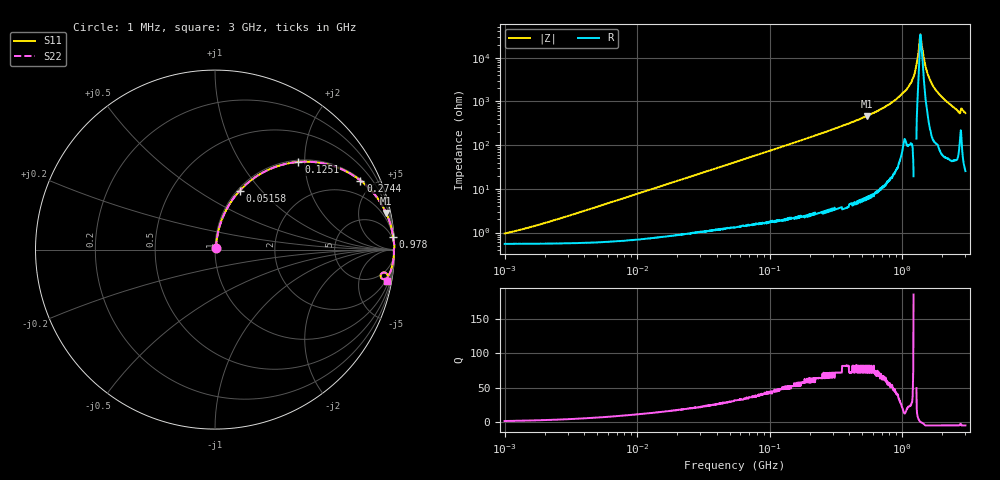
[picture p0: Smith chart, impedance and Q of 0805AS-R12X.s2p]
!s-Parameter Generated by FASTRON Sdn. Bhd.
!FASTRON P/N : 0805AS-R12X
!Keysight Technologies: E4991B_MY54100416_A.01.15
!Date: Mon Jun 15 12:52:09 2026
!Version  :Rev01  Mon Jun 15 12:52:09 2026
!Data & Calibration Information:
!Freq  S11  S21  S12  S22
!PortZ  Port1:50+j0  Port2:50+j0
!When reading reference impedance value at option line is always used.
! Remarks : This data is being provided solely for informational purposes.
# Hz S dB R 50
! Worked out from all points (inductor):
!   1601 points, 1 MHz to 3 GHz, reference 50 ohm
!   read as one part in series: L = 123 nH near 2.172 MHz
!   highest Q = 81.6 at 541.9 MHz (marker M1), where L = 137 nH
!   self-resonance near 1.374 GHz
!   S11 on the Smith chart (normalised r, x): 1 MHz: 1.01, +0.02; 51.58 MHz: 1.03, +0.77; 125.1 MHz: 1.04, +1.86; 274.4 MHz: 1.06, +4.18; 978 MHz: 2, +28; 3 GHz: 2, -11
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1000000  -40.50 54.2  -0.05 -0.4  -0.05 -0.4  -40.50 54.2
3804036  -30.50 77.2  -0.05 -1.7  -0.05 -1.7  -30.50 77.2
1.447069e7  -19.30 79.7  -0.12 -6.2  -0.12 -6.2  -19.30 79.7
5.15801e7  -8.98 67.3  -0.70 -20.8  -0.70 -20.8  -8.98 67.3
5.504702e7  -8.50 66.1  -0.78 -22.1  -0.78 -22.1  -8.50 66.1
1.250659e8  -3.42 46.4  -2.80 -42.4  -2.80 -42.4  -3.42 46.4
2.083556e8  -1.55 32.3  -5.45 -56.8  -5.45 -56.8  -1.55 32.3
2.743666e8  -0.94 25.4  -7.36 -63.8  -7.36 -63.8  -0.94 25.4
5.418594e8  -0.22 12.1  -13.60 -77.1  -13.60 -77.1  -0.22 12.1
7.925923e8  -0.08 6.7  -18.70 -82.3  -18.70 -82.3  -0.08 6.7
9.779672e8  -0.04 4.0  -23.00 -83.8  -23.00 -83.8  -0.04 4.0
1.097256e9  -0.03 2.8  -26.10 -84.4  -26.10 -84.4  -0.03 2.8
1.200675e9  -0.01 1.8  -30.20 -86.7  -30.20 -86.7  -0.01 1.8
1.268618e9  0.00 1.0  -35.30 -90.2  -35.30 -90.2  0.00 1.0
1.340405e9  -0.02 0.3  -44.80 -69.0  -44.80 -69.0  -0.02 0.3
1.381259e9  -0.03 -0.0  -49.90 12.8  -49.90 12.8  -0.03 -0.0
1.416254e9  -0.04 -0.3  -44.40 47.1  -44.40 47.1  -0.04 -0.3
1.481494e9  -0.03 -0.7  -37.70 76.3  -37.70 76.3  -0.03 -0.7
1.54974e9  -0.03 -1.3  -33.00 81.9  -33.00 81.9  -0.03 -1.3
1.75626e9  -0.04 -2.9  -26.00 83.8  -26.00 83.8  -0.04 -2.9
2.620866e9  -0.22 -9.1  -16.00 76.2  -16.00 76.2  -0.22 -9.1
3e9  -0.22 -10.3  -14.90 77.0  -14.90 77.0  -0.22 -10.3
